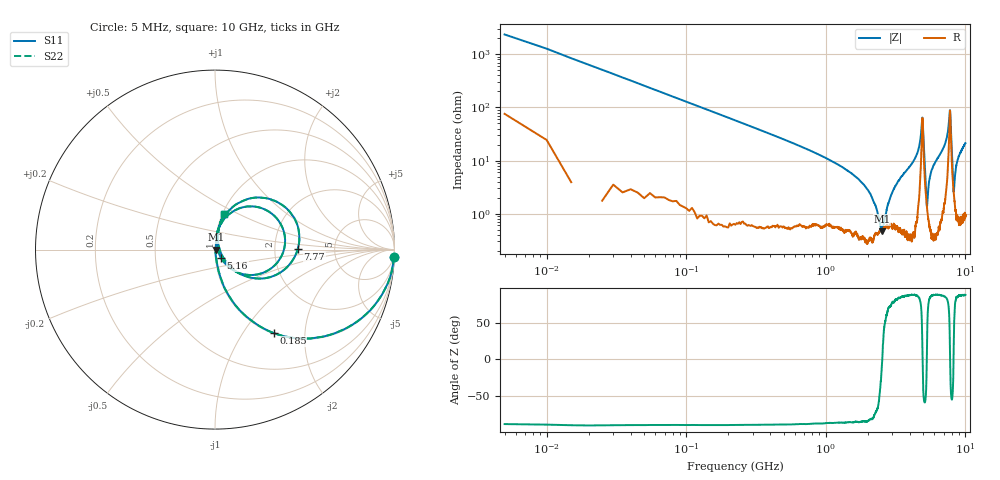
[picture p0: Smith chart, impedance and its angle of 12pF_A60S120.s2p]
! Amotech Co.,Ltd.
! http://www.amotech.co.kr/
! Part Number: A60S120
! These Parameters are Measured in Series Mode Connection
! Operation Temp=25[degC], DC Bias Voltage=0[V]
! Freq. Start=5[MHz] Stop=10[GHz], 2000[Steps]
! Date: Monday, July 13, 2020, 01:36:02
# GHZ S RI R 50.000000
!Freq.(Hz) S11(Real) S11(Imag) S21(Real) S21(Imag) S12(Real) S12(Imag) S22(Real) S22(Imag)
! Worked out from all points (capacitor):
!   2000 points, 5 MHz to 10 GHz, reference 50 ohm
!   read as one part in series: C = 12.4 pF near 55 MHz
!   lowest |Z| = 466 mohm at 2.53 GHz (marker M1)
!   series resonance near 2.539 GHz, so ESL is about 320 pH
!   S11 on the Smith chart (normalised r, x): 5 MHz: 3, -47; 185 MHz: 1.01, -1.39; 5.16 GHz: 1.06, -0.10; 7.77 GHz: 2.71, +0.02; 10 GHz: 1.02, +0.43
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0.005  0.9969 -0.0421  0.00314 0.0421  0.00314 0.0421  0.9969 -0.0421
0.08  0.7174 -0.445  0.2826 0.445  0.2826 0.445  0.7174 -0.445
0.185  0.3265 -0.4648  0.6735 0.4648  0.6735 0.4648  0.3265 -0.4648
0.515  0.0599 -0.2263  0.9401 0.2263  0.9401 0.2263  0.0599 -0.2263
1.675  0.0064 -0.0465  0.9936 0.0465  0.9936 0.0465  0.0064 -0.0465
2.53  0.00463 -0.000219  0.9954 0.000219  0.9954 0.000219  0.00463 -0.000219
2.91  0.0066 0.0196  0.9934 -0.0196  0.9934 -0.0196  0.0066 0.0196
3.34  0.00669 0.0417  0.9933 -0.0417  0.9933 -0.0417  0.00669 0.0417
4.4  0.0192 0.1126  0.9808 -0.1126  0.9808 -0.1126  0.0192 0.1126
4.825  0.1795 0.2402  0.8205 -0.2402  0.8205 -0.2402  0.1795 0.2402
5.005  0.183 -0.141  0.817 0.141  0.817 0.141  0.183 -0.141
5.16  0.0331 -0.0457  0.9669 0.0457  0.9669 0.0457  0.0331 -0.0457
5.315  0.0123 0.00612  0.9877 -0.00612  0.9877 -0.00612  0.0123 0.00612
5.7  0.0076 0.0622  0.9924 -0.0622  0.9924 -0.0622  0.0076 0.0622
6.67  0.0258 0.1346  0.9742 -0.1346  0.9742 -0.1346  0.0258 0.1346
7.595  0.2517 0.2899  0.7483 -0.2899  0.7483 -0.2899  0.2517 0.2899
7.77  0.4612 0.00325  0.5388 -0.00325  0.5388 -0.00325  0.4612 0.00325
7.885  0.2333 -0.161  0.7667 0.161  0.7667 0.161  0.2333 -0.161
8.21  0.0279 -0.00562  0.9721 0.00562  0.9721 0.00562  0.0279 -0.00562
8.335  0.0187 0.029  0.9813 -0.029  0.9813 -0.029  0.0187 0.029
8.78  0.0179 0.0991  0.9821 -0.0991  0.9821 -0.0991  0.0179 0.0991
10  0.0516 0.201  0.9484 -0.201  0.9484 -0.201  0.0516 0.201
